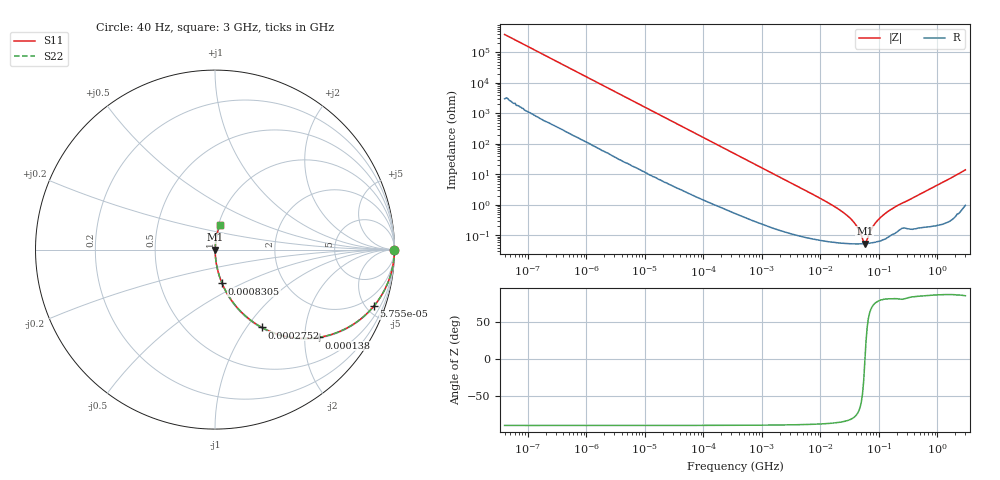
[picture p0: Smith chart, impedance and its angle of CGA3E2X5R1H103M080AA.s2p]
! S-parameter Generated by TDK Corporation
! Copyright(C) 2015 TDK Corporation.
! All Rights Reserved.
! TDK P/N: CGA3E2X5R1H103M080AA (Multilayer Ceramic Chip Capacitors)
! Property: C=10nF
! Size(LxWxT): 1.6x0.8x0.8mm, 0.063x0.031x0.031inches
! Model Type: s2p (Touchstone File Format Version 1.0)
! Frequency: DC=Yes Start=0.00004MHz Stop=3000MHz 396points Log-sweep
! Note: This model was converted from impedance.
! Model Generated on Jun. 23, 2015
! Hash(MD5):
! Port Assignments:
!  1 ---| |--- 2
! Applicable Conditions:
!  Temperature = 25 degC
!  DC Bias Voltage = 0 V
!  Small Signal Operation
! Terms and conditions regarding TDK Simulation Models
! (1)This simulation model is being provided solely for informational purposes. Please refer to the specifications of the products in terms of detailed characteristics of such products.
! (2)In no event shall TDK Corporation of any of its subsidiaries be liable for any loss or damage arising, directly or indirectly,
!  From any information contained in this simulation model, including, but not limited to loss or damages arising from any inaccuracies, omissions or errors in connection with such information.
! (3)Any and all copyrights on this simulation model are owned by TDK Corporation.
!  Duplication or redistribution of this simulation model without prior written permission from TDK Corporation is prohibited.
! (4)This simulation model is subject to any modification or change without any prior notice.
! (5)Neither TDK Corporation nor any of its subsidiaries shall make any warranty, express or implied,
!  Including but not limited to the correctness, implied warranties of merchantability and fitness for a particular purpose with respect to this simulation models.
! (6)The use of this simulation model shall be deemed to have consented to the terms and conditions hereof.
# MHz S MA R 50
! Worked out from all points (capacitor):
!   395 points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, 40 Hz to 3 GHz, reference 50 ohm
!   read as one part in series: C = 10.2 nF near 41.88 Hz
!   lowest |Z| = 53.9 mohm at 57.31 MHz (marker M1)
!   series resonance near 57.66 MHz, so ESL is about 740 pH
!   S11 on the Smith chart (normalised r, x): 40 Hz: open; 57.55 kHz: 1.05, -5.60; 138 kHz: 1.02, -2.35; 275.2 kHz: 1.01, -1.18; 830.5 kHz: 1.01, -0.39; 3 GHz: 1.02, +0.28
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4e-05  1 -0.0  0.000258 89.5  0.000258 89.5  1 -0.0
0.000834128  0.9999 -0.3  0.005282 89.3  0.005282 89.3  0.9999 -0.3
0.005256919  0.9992 -1.9  0.03297 87.7  0.03297 87.7  0.9992 -1.9
0.01739424  0.9934 -6.2  0.1079 83.4  0.1079 83.4  0.9934 -6.2
0.05755453  0.9392 -19.6  0.3356 69.9  0.3356 69.9  0.9392 -19.6
0.08708967  0.8769 -28.2  0.4731 61.3  0.4731 61.3  0.8769 -28.2
0.137988  0.7574 -40.2  0.6459 49.2  0.6459 49.2  0.7574 -40.2
0.2752031  0.5062 -59.0  0.8571 30.4  0.8571 30.4  0.5062 -59.0
0.3464102  0.4235 -64.3  0.9012 25.1  0.9012 25.1  0.4235 -64.3
0.8305245  0.193 -78.1  0.9786 11.1  0.9786 11.1  0.193 -78.1
2.084979  0.07869 -84.5  0.9955 4.5  0.9955 4.5  0.07869 -84.5
7.22376  0.02273 -86.8  0.999 1.3  0.999 1.3  0.02273 -86.8
18.13479  0.008375 -85.5  0.9994 0.5  0.9994 0.5  0.008375 -85.5
31.50375  0.003797 -81.7  0.9995 0.2  0.9995 0.2  0.003797 -81.7
43.47849  0.001756 -72.5  0.9995 0.1  0.9995 0.1  0.001756 -72.5
57.30589  0.0005391 -3.8  0.9995 0.0  0.9995 0.0  0.0005391 -3.8
60.0049  0.0005936 23.6  0.9995 -0.0  0.9995 -0.0  0.0005936 23.6
72.13343  0.001441 67.0  0.9994 -0.1  0.9994 -0.1  0.001441 67.0
86.71344  0.002531 76.3  0.9994 -0.1  0.9994 -0.1  0.002531 76.3
150.6385  0.006542 81.5  0.9991 -0.4  0.9991 -0.4  0.006542 81.5
994.0817  0.04425 84.7  0.9969 -2.5  0.9969 -2.5  0.04425 84.7
3000  0.1383 78.1  0.981 -7.9  0.981 -7.9  0.1383 78.1
